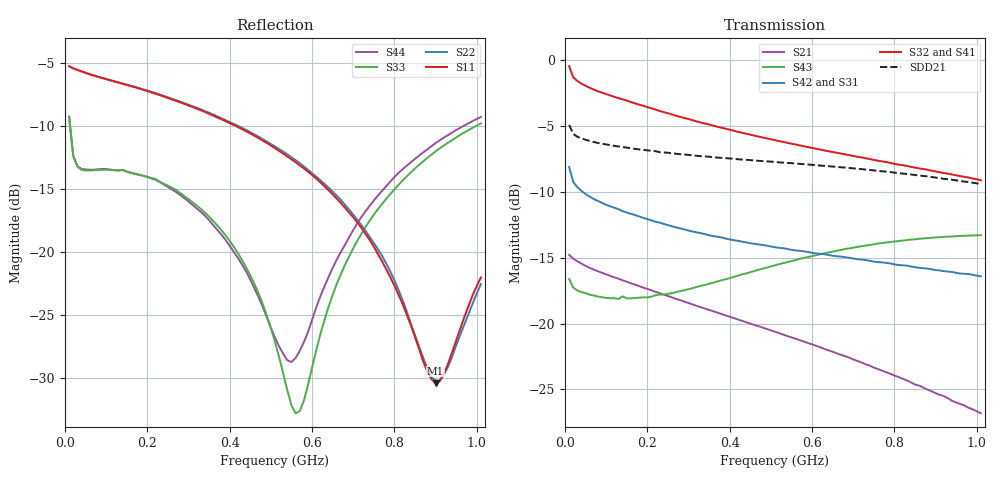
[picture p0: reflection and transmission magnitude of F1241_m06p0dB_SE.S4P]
! Integrated Device Technology
! Corporate Headquarters
! 6024 Silver Creek Valley Road
! San Jose, CA 95138  USA
! Phone:  1-408-284-8200
! Toll Free:  1-800-223-1366
! Webpage:  http://www.idt.com/
! Timing and RF Division
! 515 Groton Road, Suite 102
! Westford, MA 01886-6024
! Device:  F1241
! Description: Dual Intermediate Frequency Digital Variable Gain Amplifier
! Frequency:  10.0 -  500.00 MHz
! Package:  5x5 mm QFN Plastic Package: 32 pin
! Ports:  8 RF, 20 DC
!  Pin  1  = GA3  Pin 17  = RF OUT_B+
!  Pin  2  = GA4  Pin 18  = RF OUT_B-
!  Pin  3  = GA5  Pin 19  = STBY_B
!  Pin  4  = ISET_A  Pin 20  = Ground
!  Pin  5  = ISET_B  Pin 21  = Ground
!  Pin  6  = GB5  Pin 22  = STB_A
!  Pin  7  = GB4  Pin 23  = RF OUT_A-  = Port 4
!  Pin  8  = GB3  Pin 24  = RF OUT_A+  = Port 3
!  Pin  9  = GB2  Pin 25  = NO CONNECT
!  Pin 10  = GB1  Pin 26  = NO CONNECT
!  Pin 11  = RF IN_B+  Pin 27  = VCC
!  Pin 12  = RF IN_B-  Pin 28  = Ground
!  Pin 13  = Ground  Pin 29  = RF IN_A-  = Port 2
!  Pin 14  = VCC  Pin 30  = RF IN_A+  = Port 1
!  Pin 15  = NO CONNECT  Pin 31  = GA1
!  Pin 16  = NO CONNECT  Pin 32  = GA2
! State:  26
! Gain State:  -6.0 dB
! Voltages:  Vcc = +5.00 Volts  Icc approximately 160.0 mA or 80 mA per channel.
! Data:  The device was measured on a custom evaluation board which has
!  individual transmission lines to the RF pins.  Data was collected
!  using a calibrated network analyzer.  The evaluation board was
!  de-embedded using a port reference technique.
!  The reference plane is the edge of the package pin.
!  Only Channel A was measured.
!  This data is in single-ended operation.  If your needs are balanced
!  or differential S-parameters then this file needs to be used a
!  linear simulator.
! Misc:  Lot Code  160028MY
!  Action Tracker AT004
! Date Measured:  2014-08-14
! Date:  2014-08-28  MJV
! Note:
!  Integrated Device Technology supplies this data as a sample of measured
!  data at the package pin for this product.  Your particular data for this
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# Hz S dB R 50
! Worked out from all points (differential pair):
!   101 points, 10 MHz to 1.01 GHz, reference 50 ohm
!   strongest paths, dB at 10 MHz, 260 MHz, 510 MHz, 760 MHz, 1.01 GHz:
!     S32: -0.4, -4.1, -6.1, -7.6, -9.1
!     S41: -0.4, -4.1, -6.2, -7.8, -9.4
!     S42: -8.1, -12.6, -14.2, -15.3, -16.4
!     S31: -8.1, -12.7, -14.3, -15.5, -16.5
!     S43: -16.6, -17.7, -15.6, -13.9, -13.3
!     S21: -14.8, -18.0, -20.6, -23.5, -26.8
!   taken as a pair (ports 2,1 in; 3,4 out), SDD21 dB: -4.9, -7.1, -7.7, -8.4, -9.4
!   lowest |S11| = -30.4 dB at 900 MHz (marker M1), VSWR 1.06, Z = 52 + j2.35 ohm
!   |S11| at or under -10 dB: 412.5 MHz to end of sweep
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1e7  -5.30 -5.2  -14.77 -9.9  -33.68 -2.4  -25.34 6.5
     -14.78 -9.8  -5.29 -5.1  -25.37 6.2  -33.72 -2.3
     -8.11 157.1  -0.45 166.6  -9.35 -43.2  -16.65 178.4
     -0.40 166.7  -8.10 157.3  -16.61 178.4  -9.30 -42.9
6e7  -5.93 -8.2  -15.75 -13.7  -34.72 -8.1  -25.85 -6.3
     -15.77 -13.8  -5.93 -7.8  -25.85 -6.5  -34.78 -8.4
     -10.36 151.5  -2.09 162.6  -13.57 -9.2  -17.87 163.2
     -2.05 162.4  -10.37 151.6  -17.81 163.0  -13.51 -9.0
3.9e8  -9.65 -21.4  -19.36 -39.1  -36.43 -3.4  -27.09 -19.6
       -19.38 -39.3  -9.58 -19.8  -26.92 -19.3  -36.40 -5.3
       -13.63 75.6  -5.20 120.5  -18.72 -13.7  -16.72 107.2
       -5.27 119.2  -13.54 74.8  -16.64 106.9  -19.08 -8.7
5.6e8  -12.91 -24.3  -21.12 -46.4  -35.69 -1.1  -27.07 -25.7
       -21.16 -46.7  -12.75 -22.2  -26.72 -25.9  -35.63 -2.8
       -14.55 46.5  -6.40 103.7  -32.84 51.2  -15.29 83.4
       -6.53 102.3  -14.45 45.1  -15.18 83.1  -28.45 67.9
7e8  -17.28 -23.5  -22.66 -50.8  -34.74 -1.5  -27.06 -32.2
     -22.73 -51.2  -17.07 -21.4  -26.56 -32.5  -34.71 -4.1
     -15.20 26.0  -7.27 90.7  -19.75 126.9  -14.37 65.2
     -7.46 89.2  -15.06 23.8  -14.24 65.0  -18.30 119.7
9e8  -30.44 48.6  -25.15 -53.4  -33.41 -6.7  -27.25 -41.8
     -25.29 -53.6  -30.24 42.1  -26.49 -43.0  -33.44 -9.1
     -16.06 1.4  -8.45 72.9  -12.05 125.4  -13.62 41.8
     -8.72 71.8  -15.94 -1.8  -13.46 41.8  -11.40 121.4
1.01e9  -22.06 112.5  -26.68 -51.7  -32.78 -11.0  -27.40 -47.1
        -26.82 -51.5  -22.58 113.2  -26.51 -48.8  -32.76 -13.8
        -16.52 -10.0  -9.12 63.7  -9.84 122.5  -13.45 30.5
        -9.41 62.8  -16.41 -13.7  -13.29 30.4  -9.32 118.8
